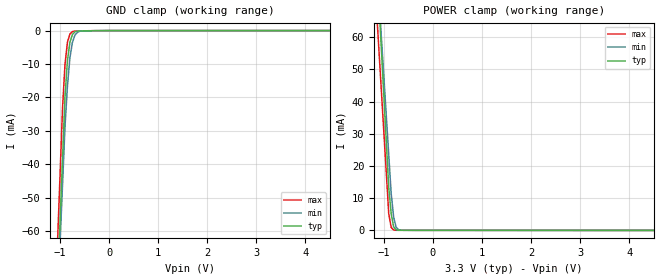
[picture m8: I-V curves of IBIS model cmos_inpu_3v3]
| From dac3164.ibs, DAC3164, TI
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[Model] cmos_inpu_3v3
Model_type Input
Vinl = 750.000mV
Vinh = 1.98000V
C_comp 865.000fF 865.000fF 865.000fF
| variable typ   min   max
[Voltage Range] 3.30000V 3.15000V 3.45000V
[POWER Clamp Reference] 3.30000V 3.15000V 3.45000V
[GND Clamp Reference] 0.00000V 0.00000V 0.00000V
[Temperature Range]   25   85   -40
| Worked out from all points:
|   GND clamp passes 1 mA (typ) near -0.74 V on its own axis
|   POWER clamp passes 1 mA (typ) near -0.80 V on its own axis
[GND Clamp]
-3.3V     -914.5mA   -858mA     -947.6mA
-950mV    -38.34mA   -45.98mA   -23.15mA
-900mV    -19.7mA    -28.71mA   -10.04mA
-850mV    -8.969mA   -16.53mA   -3.489mA
-800mV    -3.52mA    -8.174mA   -1.05mA
-750mV    -1.214mA   -3.577mA   -315uA
-700mV    -394uA     -1.426mA   -139.3uA
-650mV    -155.9uA   -568.7uA   -123.2uA
-600mV    -138uA     -195.2uA   -107.1uA
-300mV    -38.91uA   -33.85uA   -26.02uA
6.6V      0A         0A         0A
[POWER Clamp]
-3.3V     699.6mA    605.5mA    614.8mA
-1.05V    56.19mA    59.84mA    43.24mA
-900mV    13.3mA     23.47mA    5.133mA
-850mV    5.106mA    11.34mA    887.1uA
-800mV    1.082mA    4.109mA    108.8uA
-750mV    170.5uA    995.7uA    13.39uA
-700mV    25.78uA    189.9uA    11.9uA
-650mV    22.1uA     33.31uA    10.41uA
6.6V      -45.8uA    -45.48uA   -39.71uA
